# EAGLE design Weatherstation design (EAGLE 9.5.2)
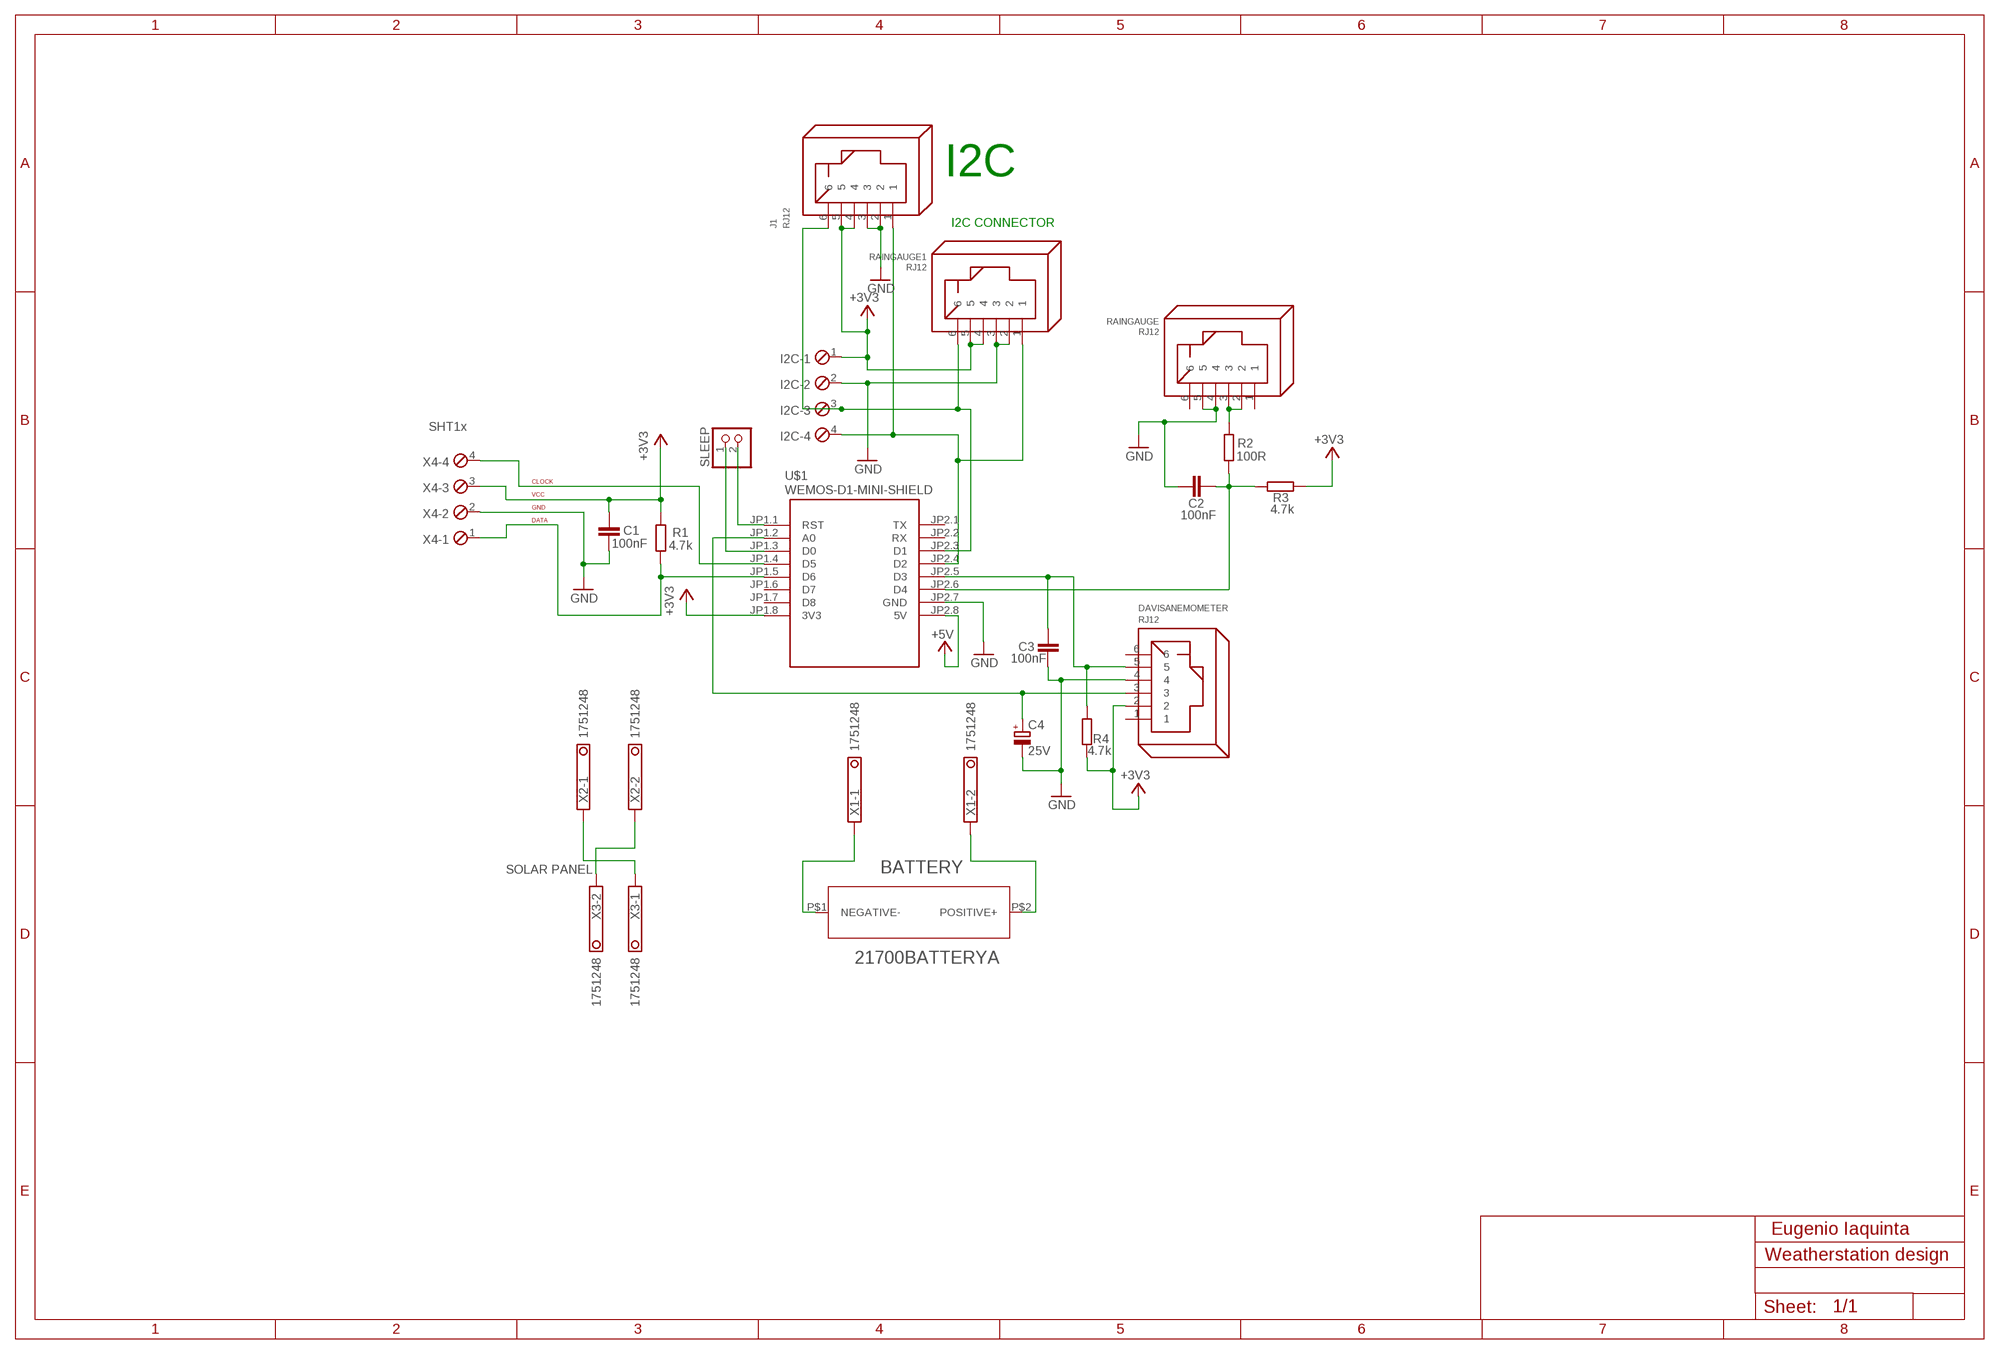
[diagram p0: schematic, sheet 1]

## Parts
BATTERY  21700BATTERYA  [21700BATTERYHOLDER]
C1  100nF  C-EUC0805  [C0805]
C2  100nF  C-EUC0805  [C0805]
C3  100nF  C-EUC0805  [C0805]
C4  25V  CPOL-EUE2.5-5  [E2,5-5]
DAVISANEMOMETER  RJ12  [RJ12]
I2C  MPT4  [4POL254]
J1  RJ12  [RJ12]
R1  4.7k  R-EU_M0805  [M0805]
R2  100R  R-EU_M0805  [M0805]
R3  4.7k  R-EU_M0805  [M0805]
R4  4.7k  R-EU_M0805  [M0805]
RAINGAUGE  RJ12  [RJ12]
RAINGAUGE1  RJ12  [RJ12]
SLEEP  PINHD-1X2  [1X02]
U$1  WEMOS-D1-MINI-SHIELD  [WEMOS-D1-MINI-SHIELD]
X1  1751248  [1751248]
X2  1751248  [1751248]
X3  1751248  [1751248]
X4  MPT4  [4POL254]

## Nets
+3V3: C1.1 DAVISANEMOMETER.2 I2C.1 J1.4 J1.5 R1.2 R3.2 R4.1 RAINGAUGE1.4 RAINGAUGE1.5 U$1.JP1.8(3V3) X4.3
+5V: U$1.JP2.8(5V)
CLOCK: U$1.JP1.4(D5) X4.4
DATA: R1.1 U$1.JP1.5(D6) X4.1
GND: C1.2 C2.1 C3.2 C4.- DAVISANEMOMETER.4 I2C.2 J1.2 J1.3 RAINGAUGE1.2 RAINGAUGE1.3 RAINGAUGE.4 RAINGAUGE.5 U$1.JP2.7(GND) X4.2
N$1: X2.2 X3.2
N$3: C2.2 R2.1 R3.1 U$1.JP2.6(D4)
N$4: R2.2 RAINGAUGE.2 RAINGAUGE.3
N$5: C4.+ DAVISANEMOMETER.3 U$1.JP1.2(A0)
N$6: C3.1 DAVISANEMOMETER.5 R4.2 U$1.JP2.5(D3)
N$7: X2.1 X3.1
N$9: SLEEP.2 U$1.JP1.1(RST)
N$10: SLEEP.1 U$1.JP1.3(D0)
NEGATIVE: BATTERY.P$1(NEGATIVE-) X1.1
POSITIVE: BATTERY.P$2(POSITIVE+) X1.2
SCL: I2C.3 J1.6 RAINGAUGE1.6 U$1.JP2.3(D1)
SDA: I2C.4 J1.1 RAINGAUGE1.1 U$1.JP2.4(D2)
Unconnected: DAVISANEMOMETER.1 DAVISANEMOMETER.6 RAINGAUGE.1 RAINGAUGE.6 U$1.JP1.6(D7) U$1.JP1.7(D8) U$1.JP2.1(TX) U$1.JP2.2(RX)

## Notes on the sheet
- I2C
- I2C CONNECTOR
- SHT1x
- CLOCK
- VCC
- GND
- DATA
- SOLAR PANEL
- Eugenio Iaquinta

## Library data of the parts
BATTERY = LithiumBatteryHolder21700:21700BATTERY
C1-C3 = rcl:C-EU: CAPACITOR, European symbol; SPICEPREFIX: C
C4 = rcl:CPOL-EU: POLARIZED CAPACITOR, European symbol; SPICEPREFIX: C
DAVISANEMOMETER J1 RAINGAUGE RAINGAUGE1 = con-rj:RJ12: RJ12, RJ14 and RJ25 RJ12, RJ14 and RJ25 jacks side mounted http://www.tycoelectronics.com
I2C X4 = con-phoenix-254:MPT4: PHOENIX CONNECTOR; OC_FARNELL: unknown; OC_NEWARK: unknown
R1-R4 = rcl:R-EU_: RESISTOR, European symbol; SPICEPREFIX: R
SLEEP = pinhead:PINHD-1X2: PIN HEADER
U$1 = diy-modules:WEMOS-D1-MINI-SHIELD: Template for WEMOS D1 mini compatible shields NOTICE: This is a template only. You can use it as a base to create symbols for WEMOS D1 mini compatible shields. Official list of available shields can be found here: https://www.wemos.cc/D1-mini-Shields
X1-X3 = con-phoenix-350:1751248: MKDS 1/ 2-3,5 Printklemme; OC_FARNELL: unknown; OC_NEWARK: unknown

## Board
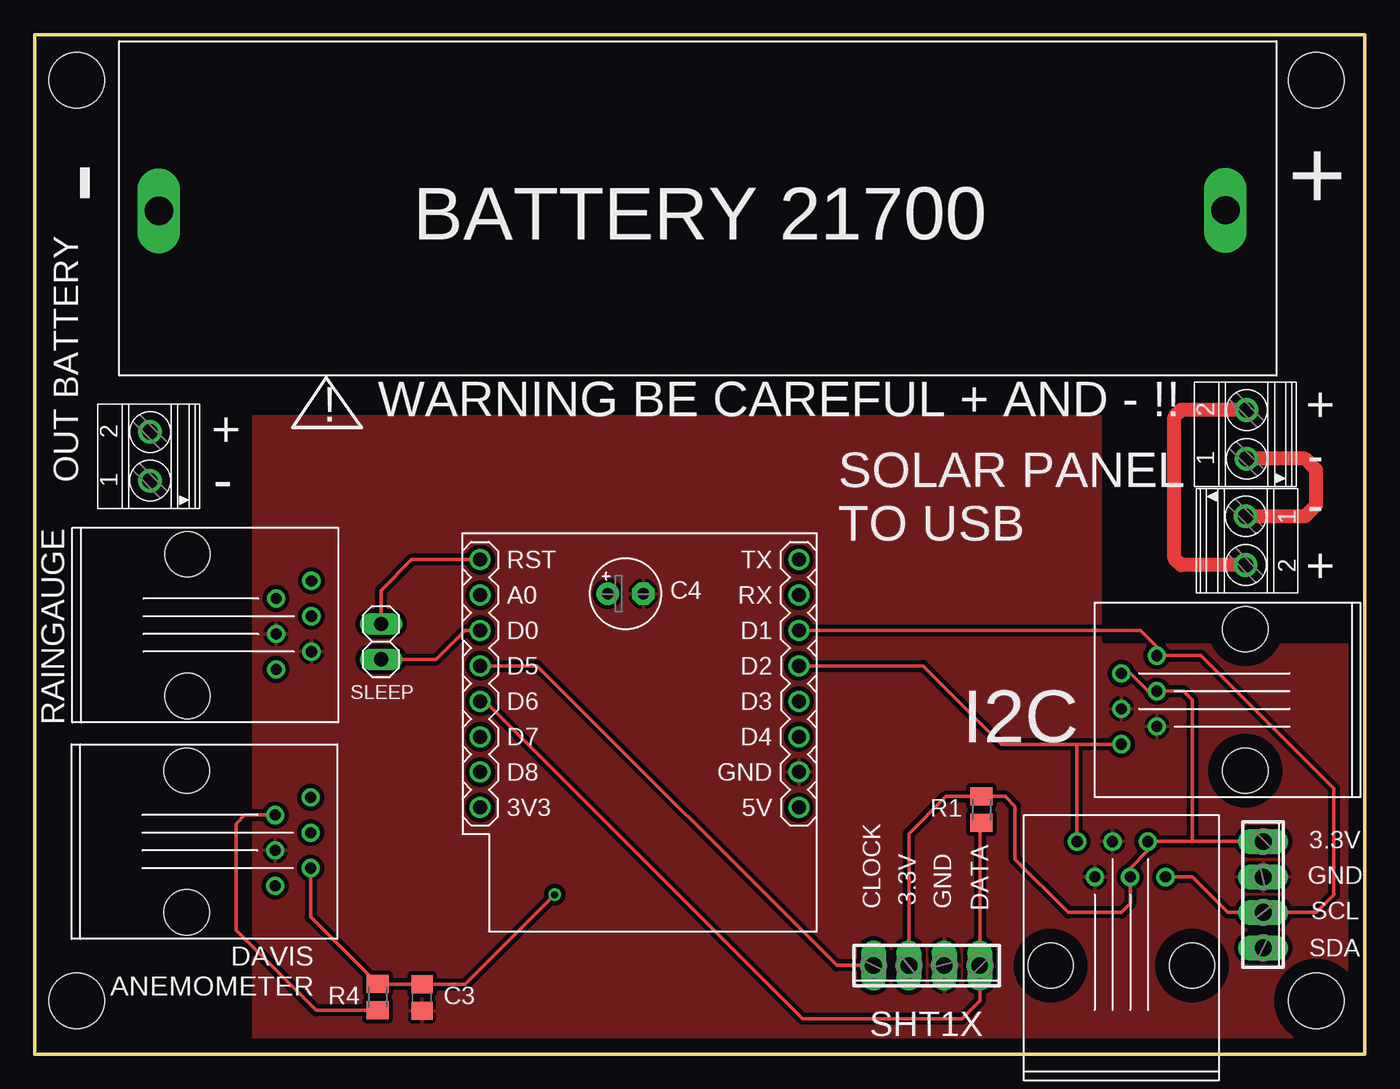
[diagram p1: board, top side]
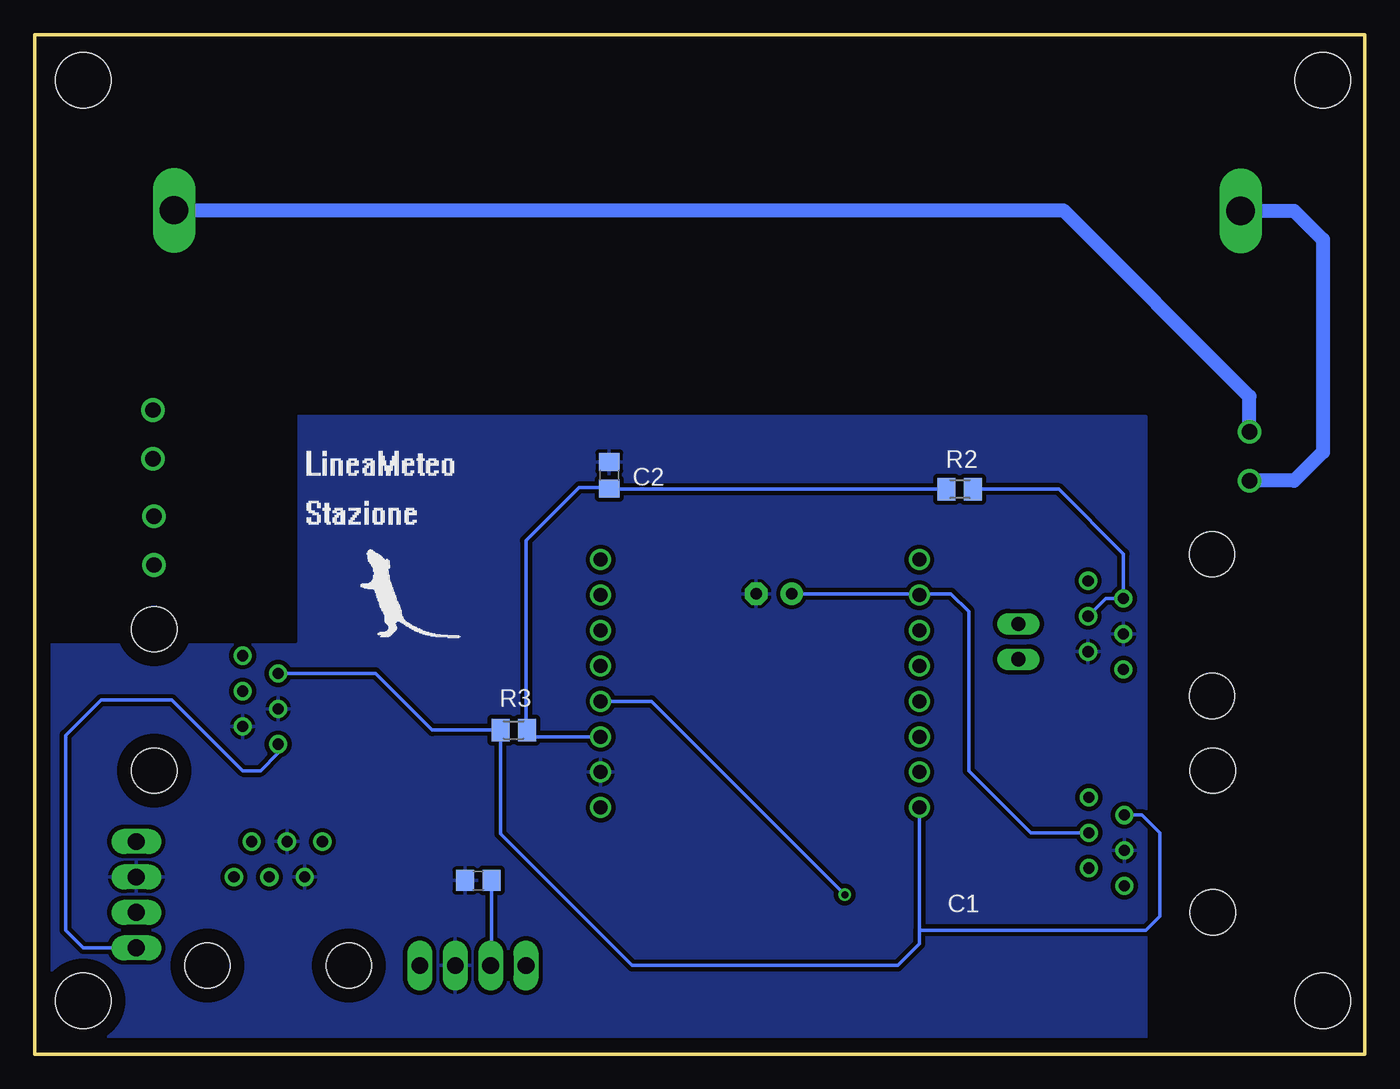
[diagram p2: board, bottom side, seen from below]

Size 95.38 x 73.11 mm. Coordinates in mm from the lower left corner, seen from the top.
Outline: 0,0 95.38,0 95.38,73.11 0,73.11 0,0
Copper layers (1*16): Top 0.035mm / dielectric 1.5mm / Bottom 0.035mm
Design rules "default": minimum track width 6mil, minimum drill 0.35mm, track to track 6mil, track to pad 6mil, pad to pad 6mil, via to via 6mil, smd to smd 6mil, copper to edge 40mil, drill to drill 6mil, minimum pad ring 10mil, minimum via ring 8mil, stop-mask expansion 4mil, vias tented up to drill 0mil, thermal gap 10mil
Holes 4 mm at 3,3.81 91.9,3.81 3,69.85 91.9,69.85

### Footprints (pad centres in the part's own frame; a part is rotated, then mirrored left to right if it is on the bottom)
21700BATTERYHOLDER = drill 2.032 long: P$1 -11.43,-0.171; P$2 65.07,-0.127
C0805 = smd 1.3 x 1.5: 1 -0.95,0; 2 0.95,0
E2,5-5 = drill 0.813 pad 1.6: + -1.27,0 | drill 0.813 pad 1.6 octagon: - 1.27,0
RJ12 = drill 0.8: 1 -8.89,-3.175; 2 -6.35,-1.905; 3 -8.89,-0.635; 4 -6.35,0.635; 5 -8.89,1.905; 6 -6.35,3.175 | hole 3.25: 0,-5.08; 0,5.08
4POL254 = drill 1.2 long: 1 -3.81,0; 2 -1.27,0; 3 1.27,0; 4 3.81,0
M0805 = smd 1.3 x 1.6: 1 -0.95,0; 2 0.95,0
1X02 = drill 1.016 long: 1 -1.27,0; 2 1.27,0
WEMOS-D1-MINI-SHIELD = drill 1: JP1.1 -11.43,12.065; JP1.2 -11.43,9.525; JP1.3 -11.43,6.985; JP1.4 -11.43,4.445; JP1.5 -11.43,1.905; JP1.6 -11.43,-0.635; JP1.7 -11.43,-3.175; JP1.8 -11.43,-5.715; JP2.1 11.43,12.065; JP2.2 11.43,9.525; JP2.3 11.43,6.985; JP2.4 11.43,4.445; JP2.5 11.43,1.905; JP2.6 11.43,-0.635; JP2.7 11.43,-3.175; JP2.8 11.43,-5.715
1751248 = drill 1.1 pad 1.7: 1 -1.75,-0.1; 2 1.75,-0.1

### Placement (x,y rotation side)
BATTERY  20.33,60.66 0 top
C1  63.58,12.45 180 bottom
C2  54.18,41.53 270 bottom
C3  27.77,4.06 270 top
C4  42.37,33.02 0 top
DAVISANEMOMETER  10.89,15.24 180 top
I2C  88.11,11.43 270 top
J1  86.82,25.4 0 top
R1  67.9,17.53 90 top
R2  29.04,40.51 0 bottom
R3  61.04,23.24 180 bottom
R4  24.59,4.08 90 top
RAINGAUGE  10.95,30.77 180 top
RAINGAUGE1  77.93,6.35 270 top
SLEEP  24.83,29.59 90 top
U$1  43.37,23.4 0 top
X1  8.16,42.88 90 top
X2  86.82,44.45 90 top
X3  86.95,36.83 270 top
X4  63.96,6.35 180 top

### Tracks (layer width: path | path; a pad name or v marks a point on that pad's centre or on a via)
+3V3
  Top 0.254: R4.1 20.19,3.13 14.43,8.89 14.43,16.51 15.07,17.14 DAVISANEMOMETER.2 | 83.01,15.24 RAINGAUGE1.5 79.84,14.61 78.56,13.33 RAINGAUGE1.4 78.56,10.79 77.93,10.16 74.12,10.16 70.31,13.97 70.31,17.78 69.61,18.48 R1.2 65.36,18.48 62.69,15.81 X4.3 | J1.5 78.56,27.3 79.84,26.04 J1.4 82.38,26.04 83.01,25.4 83.01,15.24 | 83.01,15.24 I2C.1
  Bottom 0.254: DAVISANEMOMETER.2 15.97,17.14 14.7,15.88 14.7,9.89 15.7,8.89 31.94,8.89 | J1.5 70.95,27.3 66.88,23.24 R3.2 61.99,15.81 52.53,6.35 33.48,6.35 31.94,7.89 31.94,8.89 | U$1.JP1.8 31.94,8.89 | X4.3 62.63,6.41 C1.1
CLOCK
  Top 0.254: U$1.JP1.4 36.02,27.84 57.52,6.35 X4.4
DATA
  Top 0.254: R1.1 67.77,16.45 X4.1 67.77,3.81 66.5,2.54 55.07,2.54 32.31,25.3 U$1.JP1.5
GND
  pour Top (isolate 0.305, rank 2): 95.71,45.72 15.7,45.72 15.7,0 95.71,0
  pour Bottom (isolate 0.305, rank 2): 15.7,0 95.71,0 95.71,45.72 15.7,45.72
N$1
  Top 1.016: X2.2 82.22,46.2 81.74,45.72 81.74,35.56 82.22,35.08 X3.2
N$3
  Bottom 0.254: U$1.JP2.6 59.61,22.77 59.93,23.08 R3.1 60.15,23.3 60.15,36.83 56.34,40.64 54.24,40.64 C2.2 54.11,40.51 R2.1
N$4
  Bottom 0.254: RAINGAUGE.3 18.57,32.67 RAINGAUGE.2 17.3,35.89 21.92,40.51 R2.2
N$5
  Bottom 0.254: DAVISANEMOMETER.3 23.95,15.88 28.4,20.32 28.4,31.75 29.67,33.02 31.84,33.02 U$1.JP1.2 32.03,33.02 C4.+
N$6  (via drill 0.51)
  Top 0.254: DAVISANEMOMETER.5 19.78,9.84 R4.2 24.61,5.01 C3.1 30.87,5.01 v37.29,11.43
  Bottom 0.254: U$1.JP2.5 51.17,25.3 v37.29,11.43
N$7
  Top 1.016: X3.1 91.11,38.58 91.9,39.37 91.9,41.91 91.11,42.7 X2.1
N$8
  cutout Top: 76.66,48.26 95.71,48.26 95.71,29.59 76.66,29.59
N$9
  Top 0.254: SLEEP.2 24.83,33.26 27.04,35.47 U$1.JP1.1
N$10
  Top 0.254: SLEEP.1 28.78,28.32 30.84,30.38 U$1.JP1.3
N$11
  cutout Bottom: 76.66,48.26 95.71,48.26 95.71,29.59 76.66,29.59
NEGATIVE
  Bottom 1.016: BATTERY.P$1 5.07,60.49 3,58.42 3,43.18 5.05,41.13 X1.1
POSITIVE
  Bottom 1.016: X1.2 8.26,47.17 21.62,60.53 BATTERY.P$2
SCL
  Top 0.254: RAINGAUGE1.6 83.01,12.7 85.55,10.16 88.09,10.16 I2C.3 91.9,10.16 93.17,11.43 93.17,19.05 83.64,28.57 J1.6 80.47,29.21 79.3,30.38 U$1.JP2.3
SDA
  Top 0.254: U$1.JP2.4 63.69,27.84 69.31,22.22 74.75,22.22 | RAINGAUGE1.1 74.75,22.22 | J1.1 74.75,22.22
  Bottom 0.254: J1.1 77.93,21.59 79.2,20.32 80.47,20.32 85.55,25.4 90.63,25.4 93.17,22.86 93.17,8.89 91.9,7.62 I2C.4

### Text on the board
tPlace: - | + | BATTERY 21700 | ! | WARNING BE CAREFUL + AND - !! | + | + | OUT BATTERY | - | - | - | SOLAR PANEL / TO USB | + | I2C | R1 | 3.3V | GND | CLOCK | 3.3V | GND | DATA | SCL | DAVIS / ANEMOMETER | SDA | R4 | C3 | SHT1X
bPlace: R2 | C2 | R3 | C1

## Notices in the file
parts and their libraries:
diy-modules: Released under the Creative Commons Attribution 4.0 International License: http://creativecommons.org/licenses/by/4.0
